(* Logix 5000 AddOnInstructionDefinition export Banner_Q4X_Param_v4; software revision 33.00; part 2 of 2 *)
(* tags used below, declared in another part *)
   Q4X : Banner_Q4X_v4;
   Port_Data : Banner_IOL_Port_v4;
   Port : INT;   // Enter the Port number that this AOI is to work with.
   Local_Control : DINT;
   Command_Being_Processed : BOOL;
   Update_Archive : BOOL;
   Index_Write_Inprocess : INT;
   Index_Write_Control : INT;
   Inprocess_Index : DINT;
(* Banner_Q4X_Param_v4, continued *)

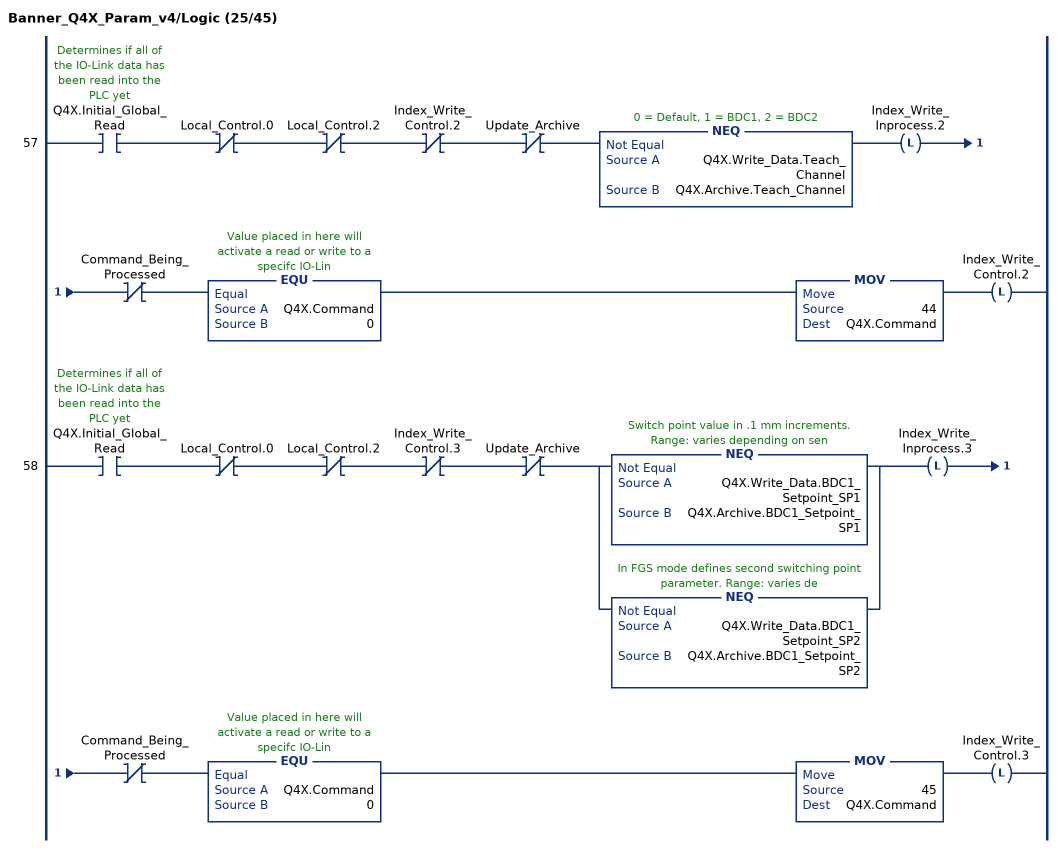
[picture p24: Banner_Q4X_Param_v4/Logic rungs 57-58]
   57: XIC(Q4X.Initial_Global_Read)XIO(Local_Control.0)XIO(Local_Control.2)XIO(Index_Write_Control.2)XIO(Update_Archive)NEQ(Q4X.Write_Data.Teach_Channel,Q4X.Archive.Teach_Channel)OTL(Index_Write_Inprocess.2)XIO(Command_Being_Processed)EQU(Q4X.Command,0)MOV(44,Q4X.Command)OTL(Index_Write_Control.2);
   58: XIC(Q4X.Initial_Global_Read)XIO(Local_Control.0)XIO(Local_Control.2)XIO(Index_Write_Control.3)XIO(Update_Archive)[NEQ(Q4X.Write_Data.BDC1_Setpoint_SP1,Q4X.Archive.BDC1_Setpoint_SP1) ,NEQ(Q4X.Write_Data.BDC1_Setpoint_SP2,Q4X.Archive.BDC1_Setpoint_SP2) ]OTL(Index_Write_Inprocess.3)XIO(Command_Being_Processed)EQU(Q4X.Command,0)MOV(45,Q4X.Command)OTL(Index_Write_Control.3);
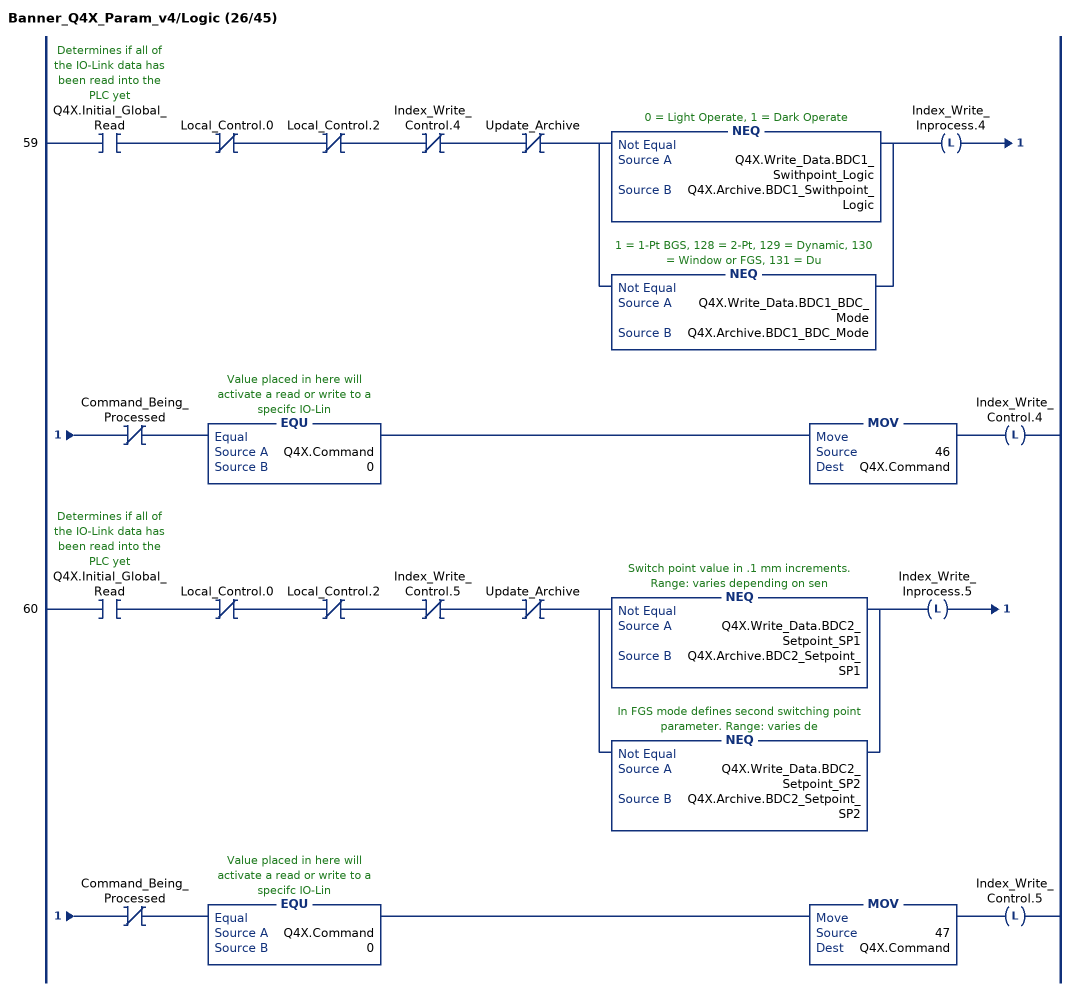
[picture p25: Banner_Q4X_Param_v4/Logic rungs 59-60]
   59: XIC(Q4X.Initial_Global_Read)XIO(Local_Control.0)XIO(Local_Control.2)XIO(Index_Write_Control.4)XIO(Update_Archive)[NEQ(Q4X.Write_Data.BDC1_Swithpoint_Logic,Q4X.Archive.BDC1_Swithpoint_Logic) ,NEQ(Q4X.Write_Data.BDC1_BDC_Mode,Q4X.Archive.BDC1_BDC_Mode) ]OTL(Index_Write_Inprocess.4)XIO(Command_Being_Processed)EQU(Q4X.Command,0)MOV(46,Q4X.Command)OTL(Index_Write_Control.4);
   60: XIC(Q4X.Initial_Global_Read)XIO(Local_Control.0)XIO(Local_Control.2)XIO(Index_Write_Control.5)XIO(Update_Archive)[NEQ(Q4X.Write_Data.BDC2_Setpoint_SP1,Q4X.Archive.BDC2_Setpoint_SP1) ,NEQ(Q4X.Write_Data.BDC2_Setpoint_SP2,Q4X.Archive.BDC2_Setpoint_SP2) ]OTL(Index_Write_Inprocess.5)XIO(Command_Being_Processed)EQU(Q4X.Command,0)MOV(47,Q4X.Command)OTL(Index_Write_Control.5);
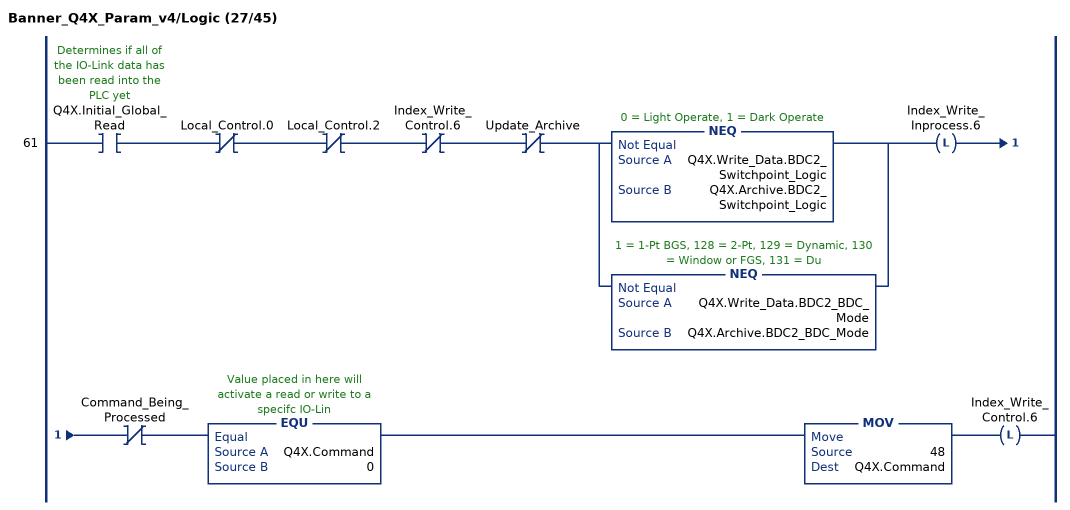
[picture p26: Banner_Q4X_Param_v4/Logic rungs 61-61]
   61: XIC(Q4X.Initial_Global_Read)XIO(Local_Control.0)XIO(Local_Control.2)XIO(Index_Write_Control.6)XIO(Update_Archive)[NEQ(Q4X.Write_Data.BDC2_Switchpoint_Logic,Q4X.Archive.BDC2_Switchpoint_Logic) ,NEQ(Q4X.Write_Data.BDC2_BDC_Mode,Q4X.Archive.BDC2_BDC_Mode) ]OTL(Index_Write_Inprocess.6)XIO(Command_Being_Processed)EQU(Q4X.Command,0)MOV(48,Q4X.Command)OTL(Index_Write_Control.6);
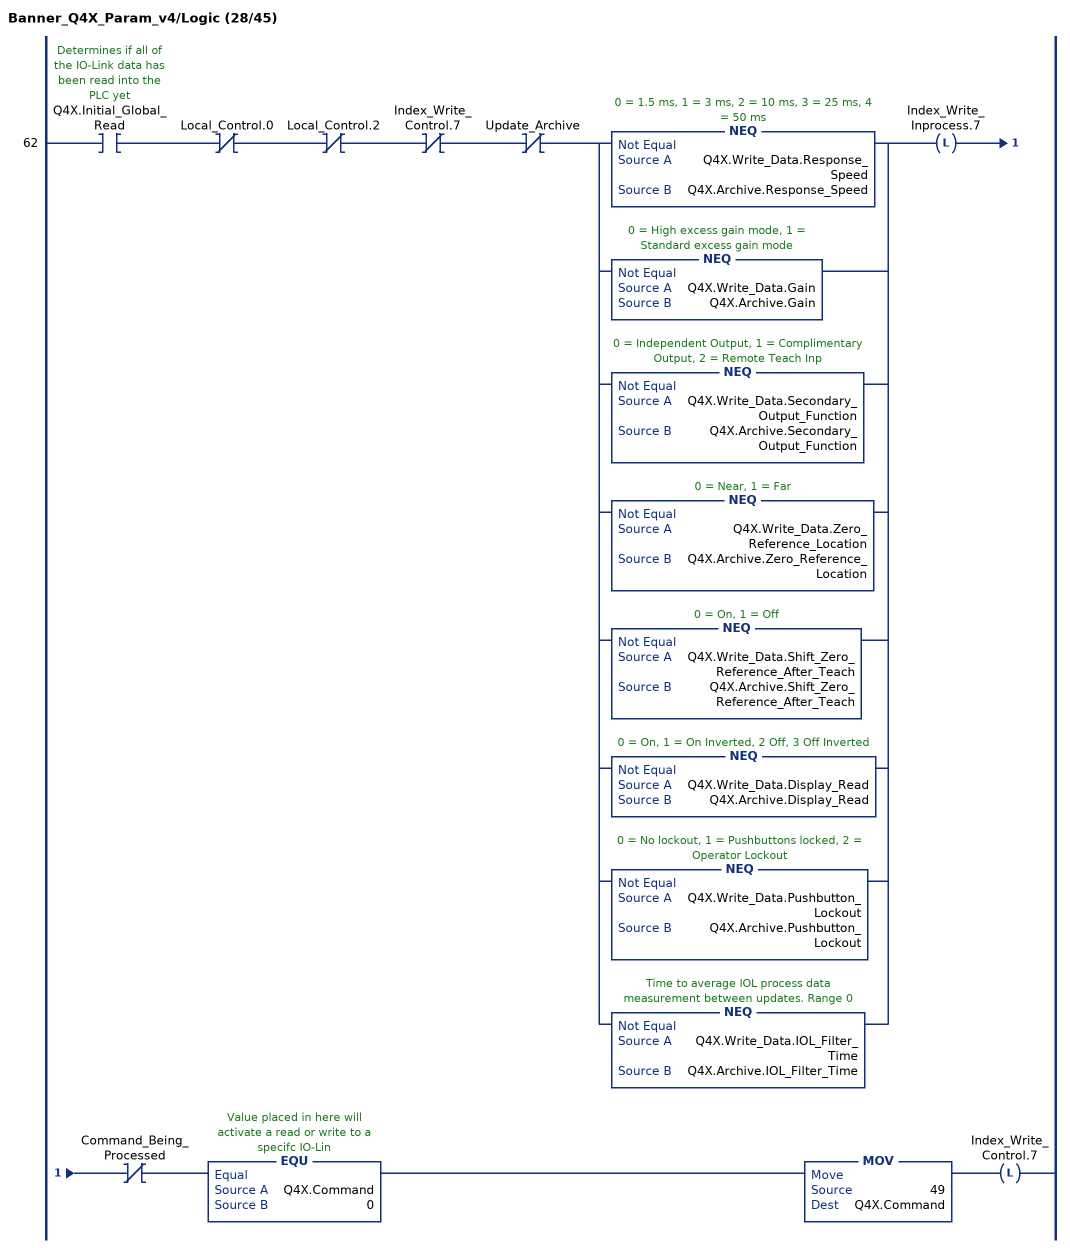
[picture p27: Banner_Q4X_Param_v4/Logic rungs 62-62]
   62: XIC(Q4X.Initial_Global_Read)XIO(Local_Control.0)XIO(Local_Control.2)XIO(Index_Write_Control.7)XIO(Update_Archive)[NEQ(Q4X.Write_Data.Response_Speed,Q4X.Archive.Response_Speed) ,NEQ(Q4X.Write_Data.Gain,Q4X.Archive.Gain) ,NEQ(Q4X.Write_Data.Secondary_Output_Function,Q4X.Archive.Secondary_Output_Function) ,NEQ(Q4X.Write_Data.Zero_Reference_Location,Q4X.Archive.Zero_Reference_Location) ,NEQ(Q4X.Write_Data.Shift_Zero_Reference_After_Teach,Q4X.Archive.Shift_Zero_Reference_After_Teach) ,NEQ(Q4X.Write_Data.Display_Read,Q4X.Archive.Display_Read) ,NEQ(Q4X.Write_Data.Pushbutton_Lockout,Q4X.Archive.Pushbutton_Lockout) ,NEQ(Q4X.Write_Data.IOL_Filter_Time,Q4X.Archive.IOL_Filter_Time) ]OTL(Index_Write_Inprocess.7)XIO(Command_Being_Processed)EQU(Q4X.Command,0)MOV(49,Q4X.Command)OTL(Index_Write_Control.7);
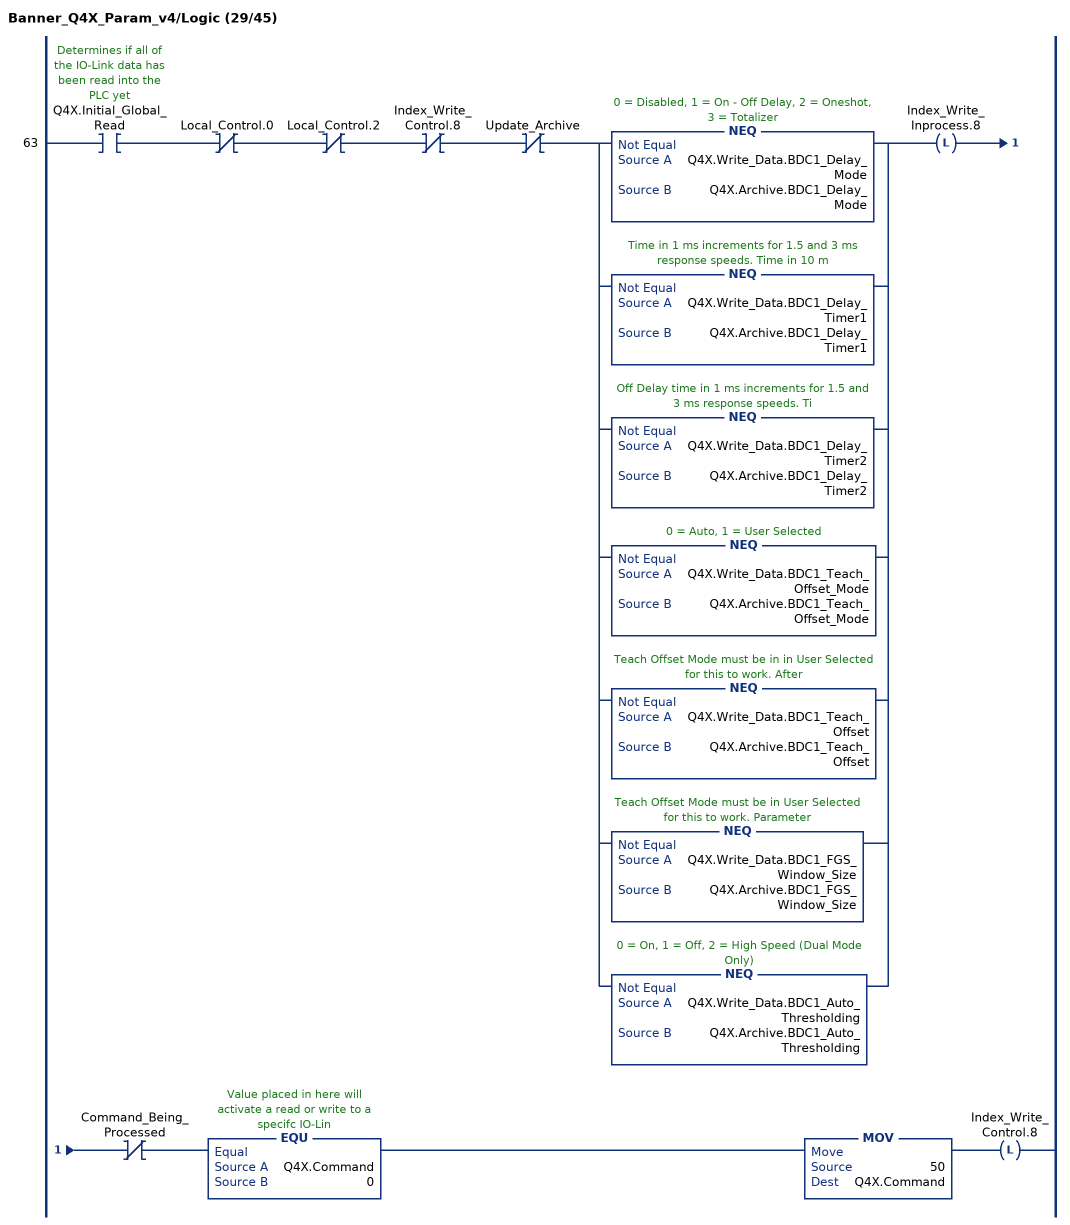
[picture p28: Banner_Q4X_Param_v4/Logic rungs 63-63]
   63: XIC(Q4X.Initial_Global_Read)XIO(Local_Control.0)XIO(Local_Control.2)XIO(Index_Write_Control.8)XIO(Update_Archive)[NEQ(Q4X.Write_Data.BDC1_Delay_Mode,Q4X.Archive.BDC1_Delay_Mode) ,NEQ(Q4X.Write_Data.BDC1_Delay_Timer1,Q4X.Archive.BDC1_Delay_Timer1) ,NEQ(Q4X.Write_Data.BDC1_Delay_Timer2,Q4X.Archive.BDC1_Delay_Timer2) ,NEQ(Q4X.Write_Data.BDC1_Teach_Offset_Mode,Q4X.Archive.BDC1_Teach_Offset_Mode) ,NEQ(Q4X.Write_Data.BDC1_Teach_Offset,Q4X.Archive.BDC1_Teach_Offset) ,NEQ(Q4X.Write_Data.BDC1_FGS_Window_Size,Q4X.Archive.BDC1_FGS_Window_Size) ,NEQ(Q4X.Write_Data.BDC1_Auto_Thresholding,Q4X.Archive.BDC1_Auto_Thresholding) ]OTL(Index_Write_Inprocess.8)XIO(Command_Being_Processed)EQU(Q4X.Command,0)MOV(50,Q4X.Command)OTL(Index_Write_Control.8);
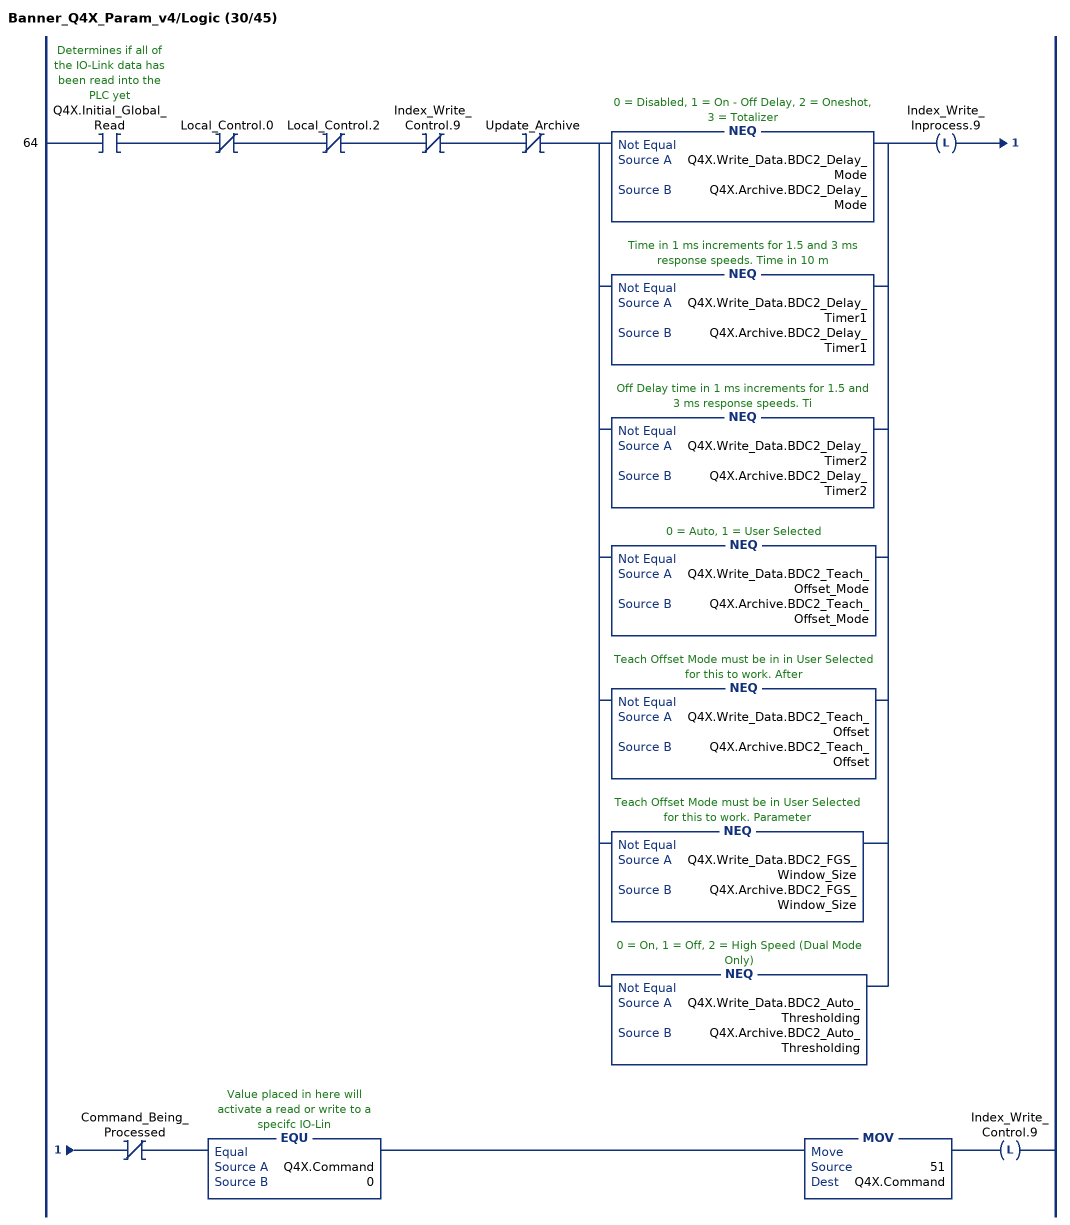
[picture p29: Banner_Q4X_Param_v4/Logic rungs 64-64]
   64: XIC(Q4X.Initial_Global_Read)XIO(Local_Control.0)XIO(Local_Control.2)XIO(Index_Write_Control.9)XIO(Update_Archive)[NEQ(Q4X.Write_Data.BDC2_Delay_Mode,Q4X.Archive.BDC2_Delay_Mode) ,NEQ(Q4X.Write_Data.BDC2_Delay_Timer1,Q4X.Archive.BDC2_Delay_Timer1) ,NEQ(Q4X.Write_Data.BDC2_Delay_Timer2,Q4X.Archive.BDC2_Delay_Timer2) ,NEQ(Q4X.Write_Data.BDC2_Teach_Offset_Mode,Q4X.Archive.BDC2_Teach_Offset_Mode) ,NEQ(Q4X.Write_Data.BDC2_Teach_Offset,Q4X.Archive.BDC2_Teach_Offset) ,NEQ(Q4X.Write_Data.BDC2_FGS_Window_Size,Q4X.Archive.BDC2_FGS_Window_Size) ,NEQ(Q4X.Write_Data.BDC2_Auto_Thresholding,Q4X.Archive.BDC2_Auto_Thresholding) ]OTL(Index_Write_Inprocess.9)XIO(Command_Being_Processed)EQU(Q4X.Command,0)MOV(51,Q4X.Command)OTL(Index_Write_Control.9);
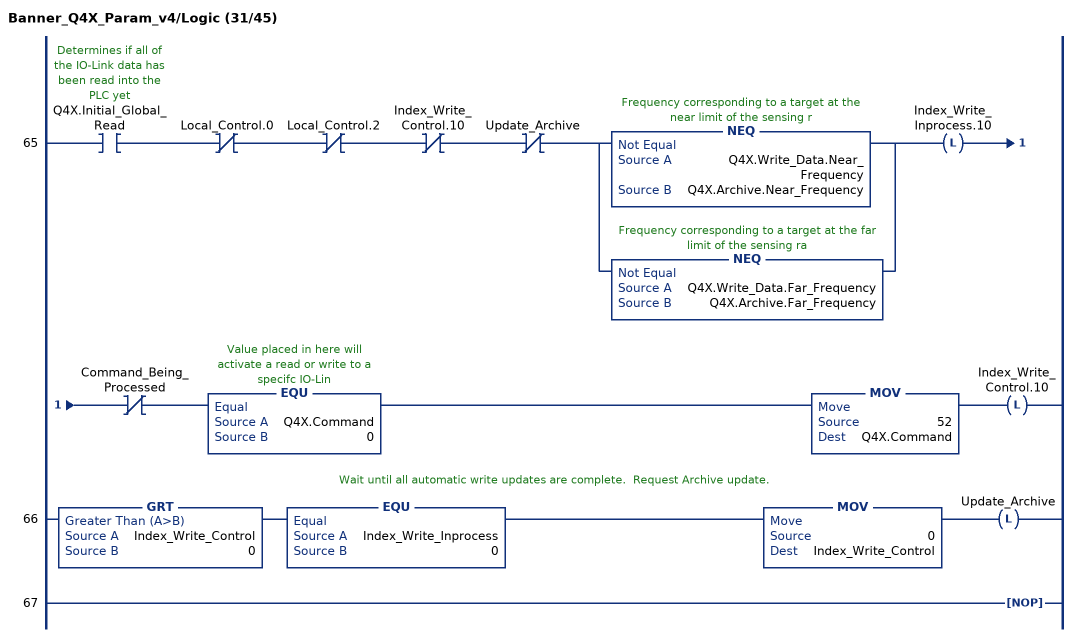
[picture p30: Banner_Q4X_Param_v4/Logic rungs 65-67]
   65: XIC(Q4X.Initial_Global_Read)XIO(Local_Control.0)XIO(Local_Control.2)XIO(Index_Write_Control.10)XIO(Update_Archive)[NEQ(Q4X.Write_Data.Near_Frequency,Q4X.Archive.Near_Frequency) ,NEQ(Q4X.Write_Data.Far_Frequency,Q4X.Archive.Far_Frequency) ]OTL(Index_Write_Inprocess.10)XIO(Command_Being_Processed)EQU(Q4X.Command,0)MOV(52,Q4X.Command)OTL(Index_Write_Control.10);
   // Wait until all automatic write updates are complete.  Request Archive update.
   66: GRT(Index_Write_Control,0)EQU(Index_Write_Inprocess,0)MOV(0,Index_Write_Control)OTL(Update_Archive);
   67: NOP();
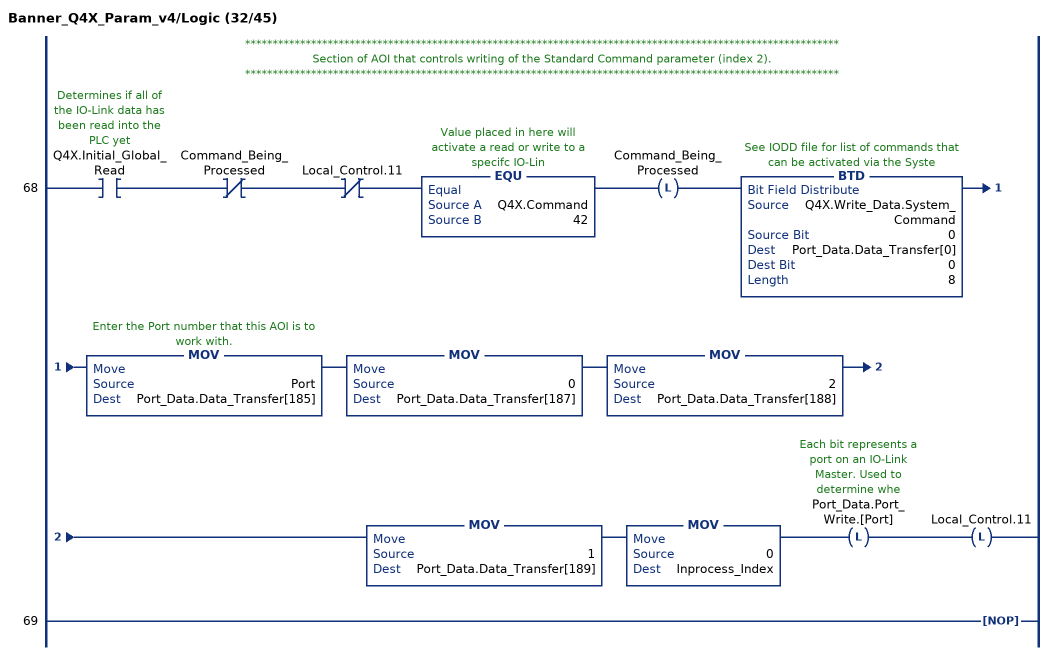
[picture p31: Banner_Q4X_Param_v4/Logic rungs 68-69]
   // ************************************************************************************************************
   // Section of AOI that controls writing of the Standard Command parameter (index 2).
   // ************************************************************************************************************
   68: XIC(Q4X.Initial_Global_Read)XIO(Command_Being_Processed)XIO(Local_Control.11)EQU(Q4X.Command,42)OTL(Command_Being_Processed)BTD(Q4X.Write_Data.System_Command,0,Port_Data.Data_Transfer[0],0,8)MOV(Port,Port_Data.Data_Transfer[185])MOV(0,Port_Data.Data_Transfer[187])MOV(2,Port_Data.Data_Transfer[188])MOV(1,Port_Data.Data_Transfer[189])MOV(0,Inprocess_Index)OTL(Port_Data.Port_Write.[Port])OTL(Local_Control.11);
   69: NOP();
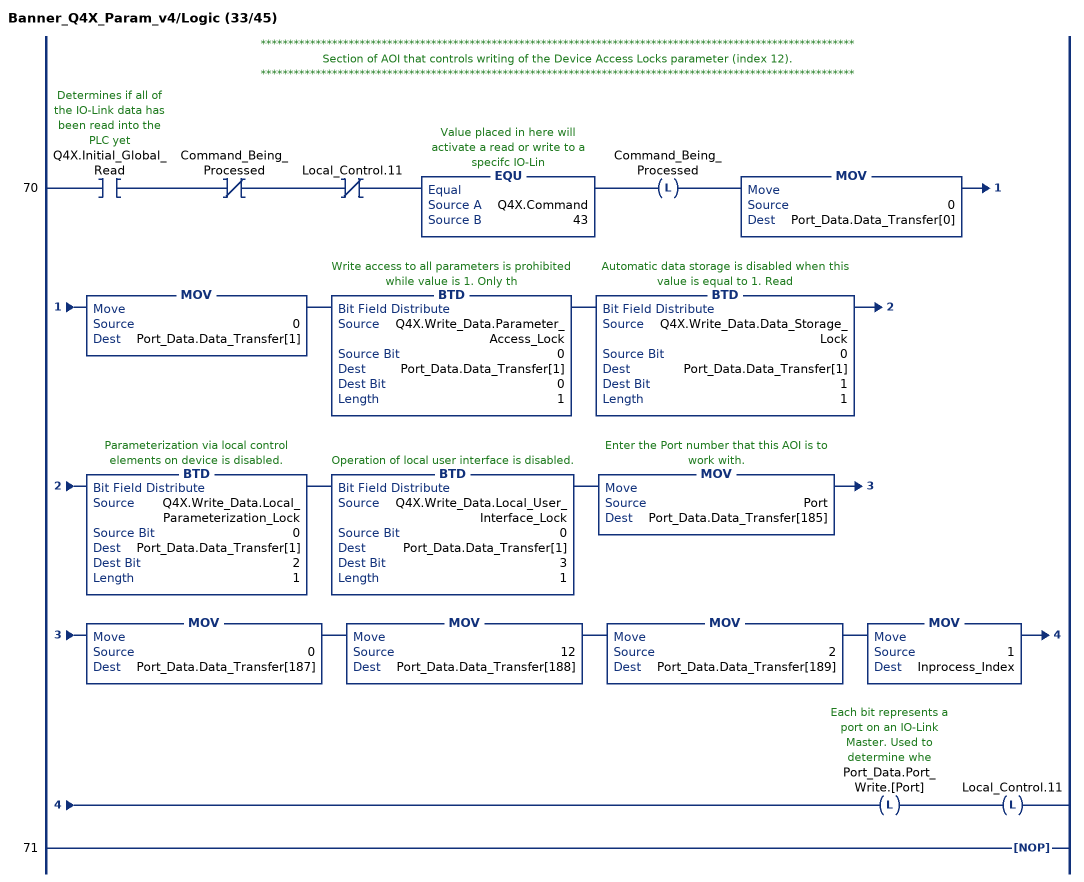
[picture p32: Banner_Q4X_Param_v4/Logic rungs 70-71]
   // ************************************************************************************************************
   // Section of AOI that controls writing of the Device Access Locks parameter (index 12).
   // ************************************************************************************************************
   70: XIC(Q4X.Initial_Global_Read)XIO(Command_Being_Processed)XIO(Local_Control.11)EQU(Q4X.Command,43)OTL(Command_Being_Processed)MOV(0,Port_Data.Data_Transfer[0])MOV(0,Port_Data.Data_Transfer[1])BTD(Q4X.Write_Data.Parameter_Access_Lock,0,Port_Data.Data_Transfer[1],0,1)BTD(Q4X.Write_Data.Data_Storage_Lock,0,Port_Data.Data_Transfer[1],1,1)BTD(Q4X.Write_Data.Local_Parameterization_Lock,0,Port_Data.Data_Transfer[1],2,1)BTD(Q4X.Write_Data.Local_User_Interface_Lock,0,Port_Data.Data_Transfer[1],3,1)MOV(Port,Port_Data.Data_Transfer[185])MOV(0,Port_Data.Data_Transfer[187])MOV(12,Port_Data.Data_Transfer[188])MOV(2,Port_Data.Data_Transfer[189])MOV(1,Inprocess_Index)OTL(Port_Data.Port_Write.[Port])OTL(Local_Control.11);
   71: NOP();
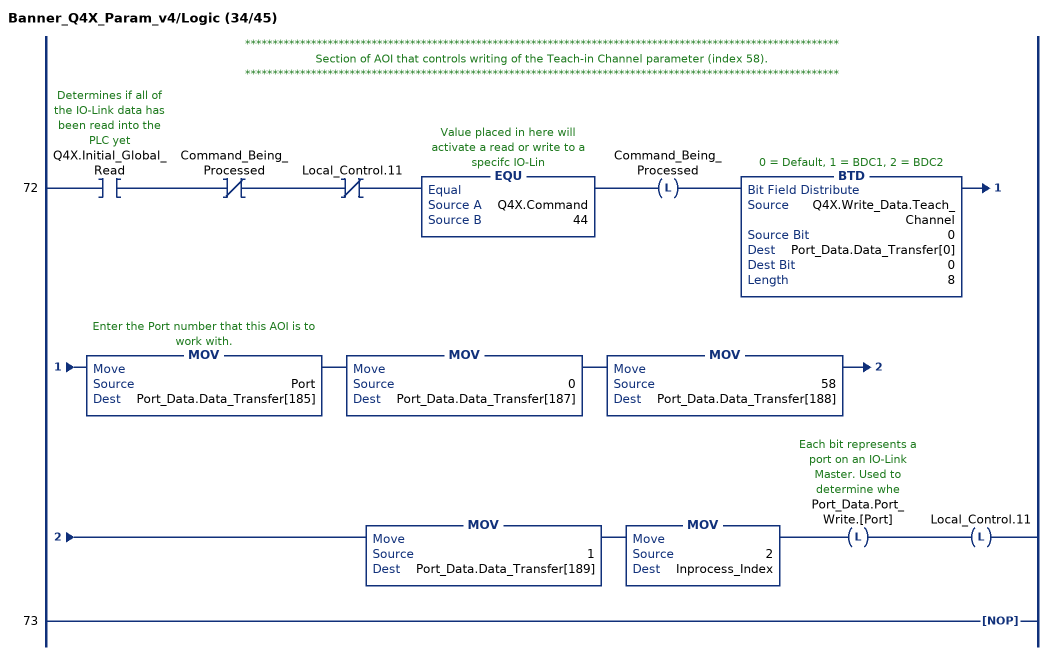
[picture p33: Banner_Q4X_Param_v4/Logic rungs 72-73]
   // ************************************************************************************************************
   // Section of AOI that controls writing of the Teach-in Channel parameter (index 58).
   // ************************************************************************************************************
   72: XIC(Q4X.Initial_Global_Read)XIO(Command_Being_Processed)XIO(Local_Control.11)EQU(Q4X.Command,44)OTL(Command_Being_Processed)BTD(Q4X.Write_Data.Teach_Channel,0,Port_Data.Data_Transfer[0],0,8)MOV(Port,Port_Data.Data_Transfer[185])MOV(0,Port_Data.Data_Transfer[187])MOV(58,Port_Data.Data_Transfer[188])MOV(1,Port_Data.Data_Transfer[189])MOV(2,Inprocess_Index)OTL(Port_Data.Port_Write.[Port])OTL(Local_Control.11);
   73: NOP();
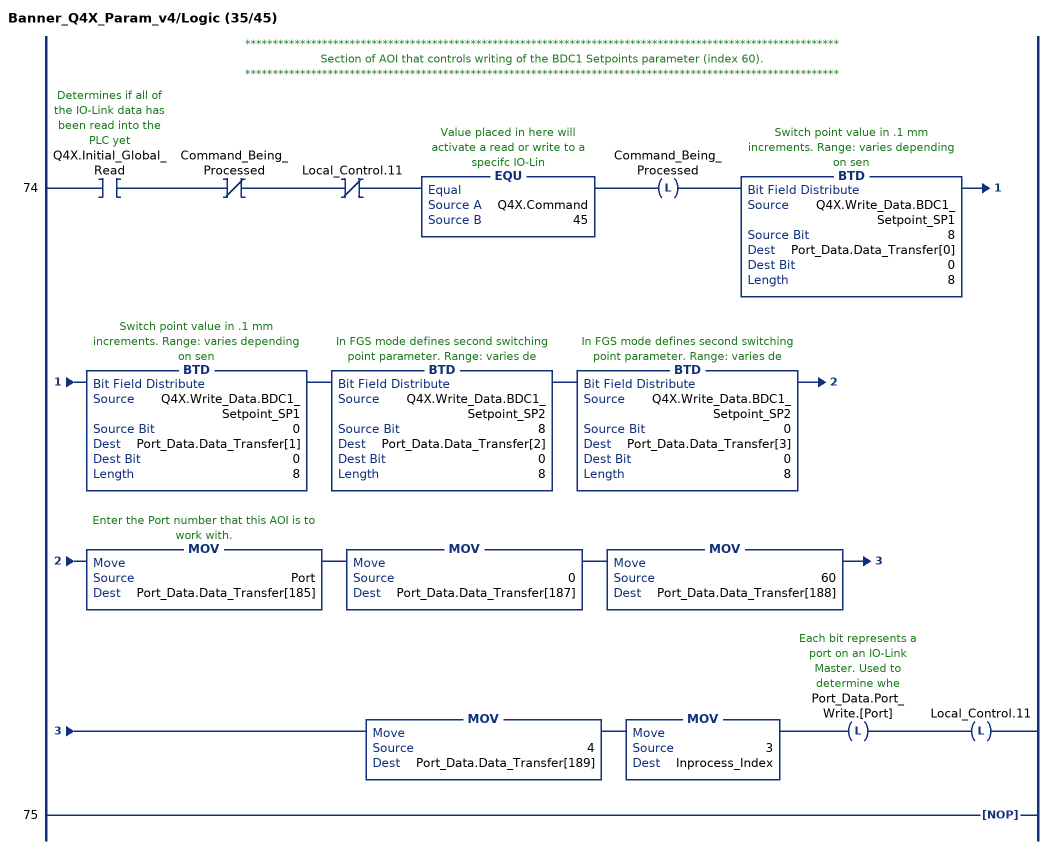
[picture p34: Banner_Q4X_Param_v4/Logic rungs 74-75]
   // ************************************************************************************************************
   // Section of AOI that controls writing of the BDC1 Setpoints parameter (index 60).
   // ************************************************************************************************************
   74: XIC(Q4X.Initial_Global_Read)XIO(Command_Being_Processed)XIO(Local_Control.11)EQU(Q4X.Command,45)OTL(Command_Being_Processed)BTD(Q4X.Write_Data.BDC1_Setpoint_SP1,8,Port_Data.Data_Transfer[0],0,8)BTD(Q4X.Write_Data.BDC1_Setpoint_SP1,0,Port_Data.Data_Transfer[1],0,8)BTD(Q4X.Write_Data.BDC1_Setpoint_SP2,8,Port_Data.Data_Transfer[2],0,8)BTD(Q4X.Write_Data.BDC1_Setpoint_SP2,0,Port_Data.Data_Transfer[3],0,8)MOV(Port,Port_Data.Data_Transfer[185])MOV(0,Port_Data.Data_Transfer[187])MOV(60,Port_Data.Data_Transfer[188])MOV(4,Port_Data.Data_Transfer[189])MOV(3,Inprocess_Index)OTL(Port_Data.Port_Write.[Port])OTL(Local_Control.11);
   75: NOP();
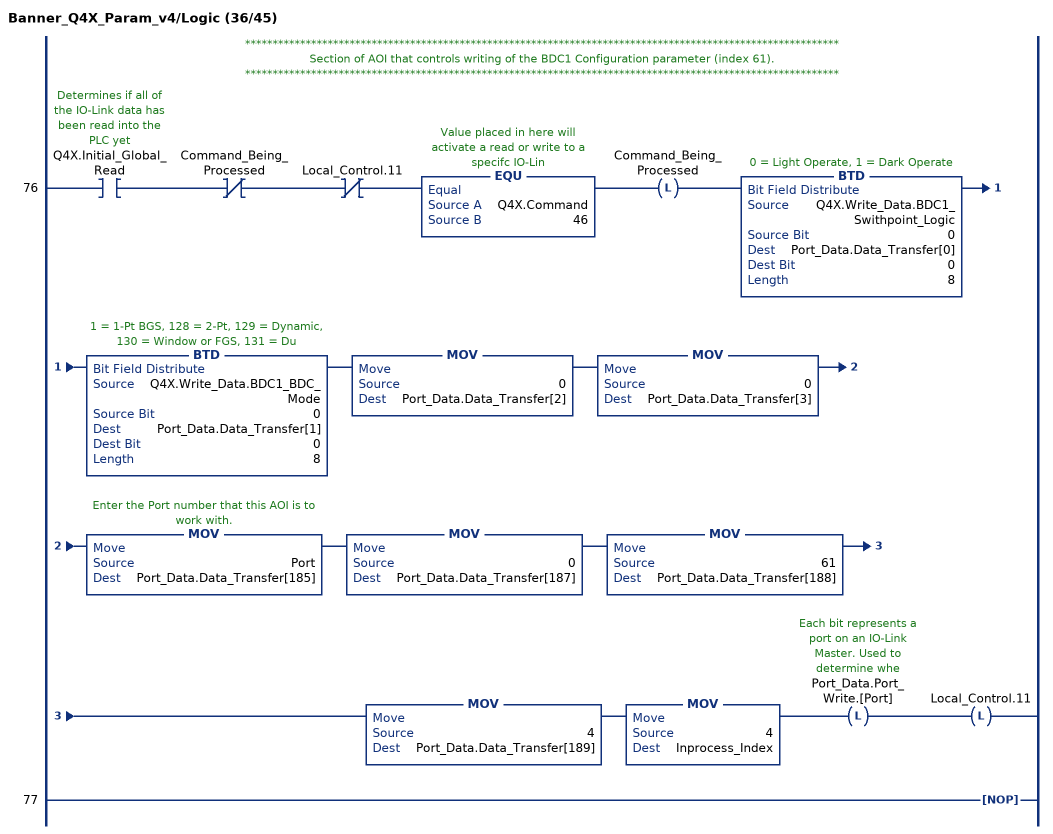
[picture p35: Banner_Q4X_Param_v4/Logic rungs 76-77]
   // ************************************************************************************************************
   // Section of AOI that controls writing of the BDC1 Configuration parameter (index 61).
   // ************************************************************************************************************
   76: XIC(Q4X.Initial_Global_Read)XIO(Command_Being_Processed)XIO(Local_Control.11)EQU(Q4X.Command,46)OTL(Command_Being_Processed)BTD(Q4X.Write_Data.BDC1_Swithpoint_Logic,0,Port_Data.Data_Transfer[0],0,8)BTD(Q4X.Write_Data.BDC1_BDC_Mode,0,Port_Data.Data_Transfer[1],0,8)MOV(0,Port_Data.Data_Transfer[2])MOV(0,Port_Data.Data_Transfer[3])MOV(Port,Port_Data.Data_Transfer[185])MOV(0,Port_Data.Data_Transfer[187])MOV(61,Port_Data.Data_Transfer[188])MOV(4,Port_Data.Data_Transfer[189])MOV(4,Inprocess_Index)OTL(Port_Data.Port_Write.[Port])OTL(Local_Control.11);
   77: NOP();
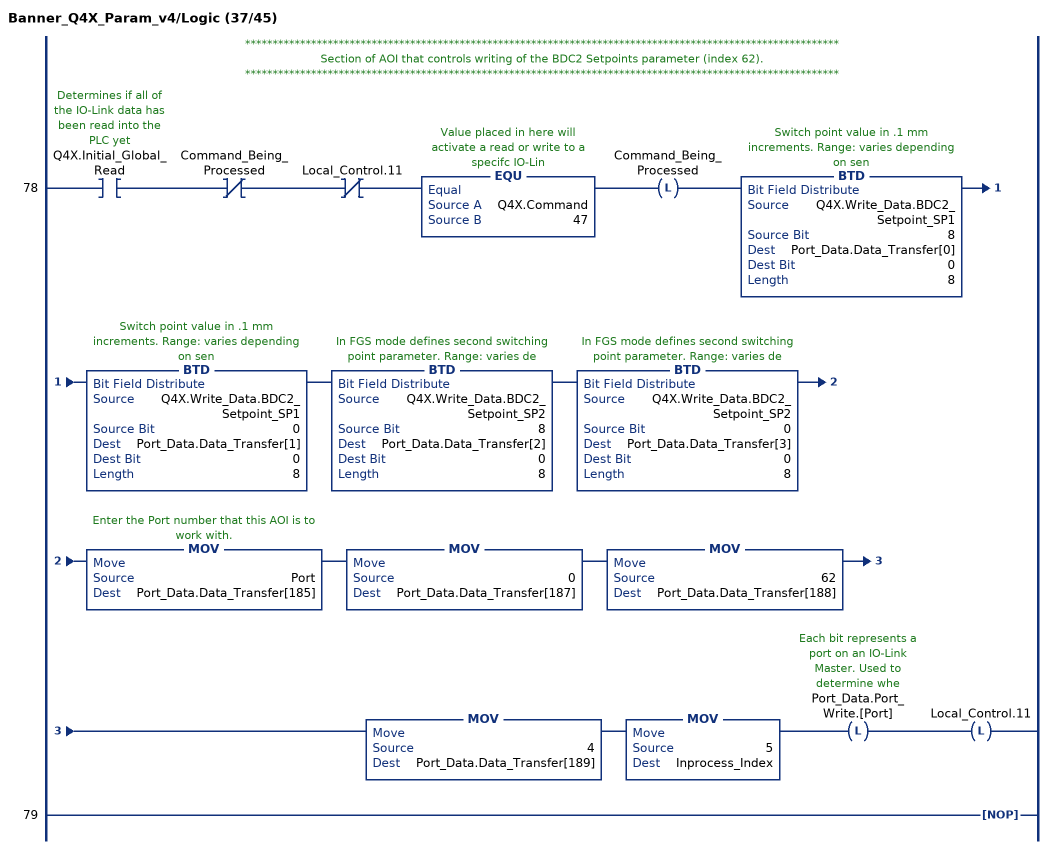
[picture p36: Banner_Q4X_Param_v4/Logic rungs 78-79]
   // ************************************************************************************************************
   // Section of AOI that controls writing of the BDC2 Setpoints parameter (index 62).
   // ************************************************************************************************************
   78: XIC(Q4X.Initial_Global_Read)XIO(Command_Being_Processed)XIO(Local_Control.11)EQU(Q4X.Command,47)OTL(Command_Being_Processed)BTD(Q4X.Write_Data.BDC2_Setpoint_SP1,8,Port_Data.Data_Transfer[0],0,8)BTD(Q4X.Write_Data.BDC2_Setpoint_SP1,0,Port_Data.Data_Transfer[1],0,8)BTD(Q4X.Write_Data.BDC2_Setpoint_SP2,8,Port_Data.Data_Transfer[2],0,8)BTD(Q4X.Write_Data.BDC2_Setpoint_SP2,0,Port_Data.Data_Transfer[3],0,8)MOV(Port,Port_Data.Data_Transfer[185])MOV(0,Port_Data.Data_Transfer[187])MOV(62,Port_Data.Data_Transfer[188])MOV(4,Port_Data.Data_Transfer[189])MOV(5,Inprocess_Index)OTL(Port_Data.Port_Write.[Port])OTL(Local_Control.11);
   79: NOP();
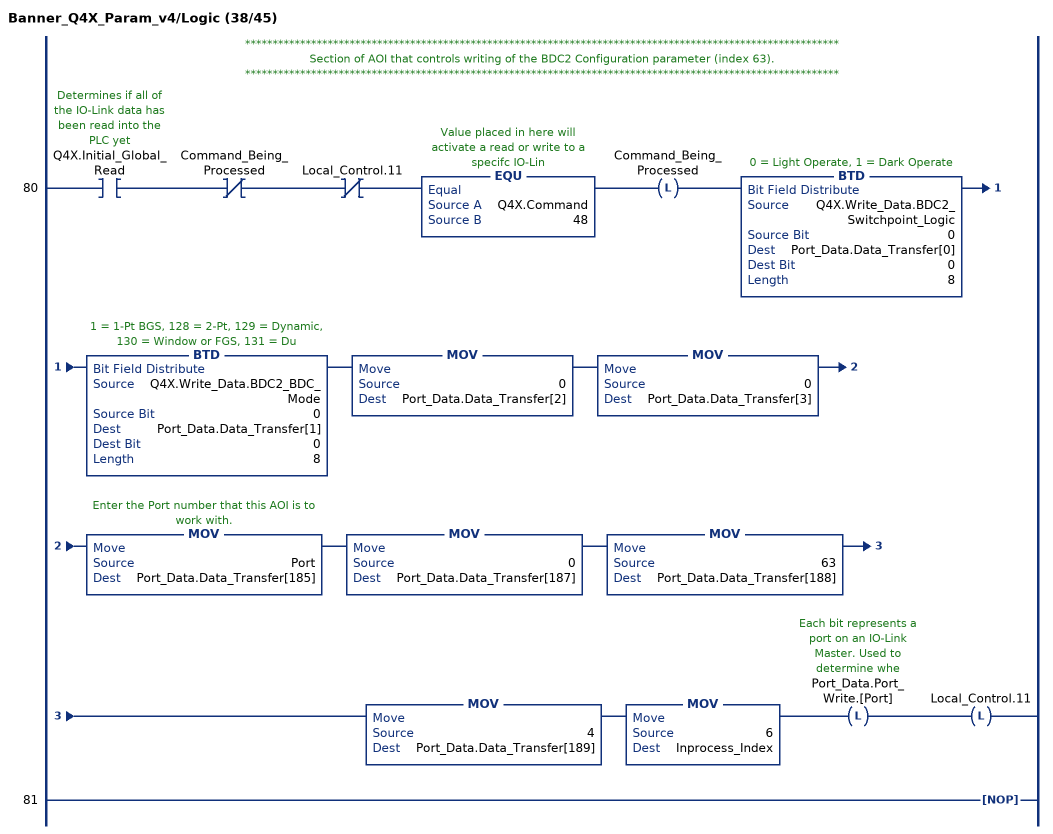
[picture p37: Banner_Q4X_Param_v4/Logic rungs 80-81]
   // ************************************************************************************************************
   // Section of AOI that controls writing of the BDC2 Configuration parameter (index 63).
   // ************************************************************************************************************
   80: XIC(Q4X.Initial_Global_Read)XIO(Command_Being_Processed)XIO(Local_Control.11)EQU(Q4X.Command,48)OTL(Command_Being_Processed)BTD(Q4X.Write_Data.BDC2_Switchpoint_Logic,0,Port_Data.Data_Transfer[0],0,8)BTD(Q4X.Write_Data.BDC2_BDC_Mode,0,Port_Data.Data_Transfer[1],0,8)MOV(0,Port_Data.Data_Transfer[2])MOV(0,Port_Data.Data_Transfer[3])MOV(Port,Port_Data.Data_Transfer[185])MOV(0,Port_Data.Data_Transfer[187])MOV(63,Port_Data.Data_Transfer[188])MOV(4,Port_Data.Data_Transfer[189])MOV(6,Inprocess_Index)OTL(Port_Data.Port_Write.[Port])OTL(Local_Control.11);
   81: NOP();
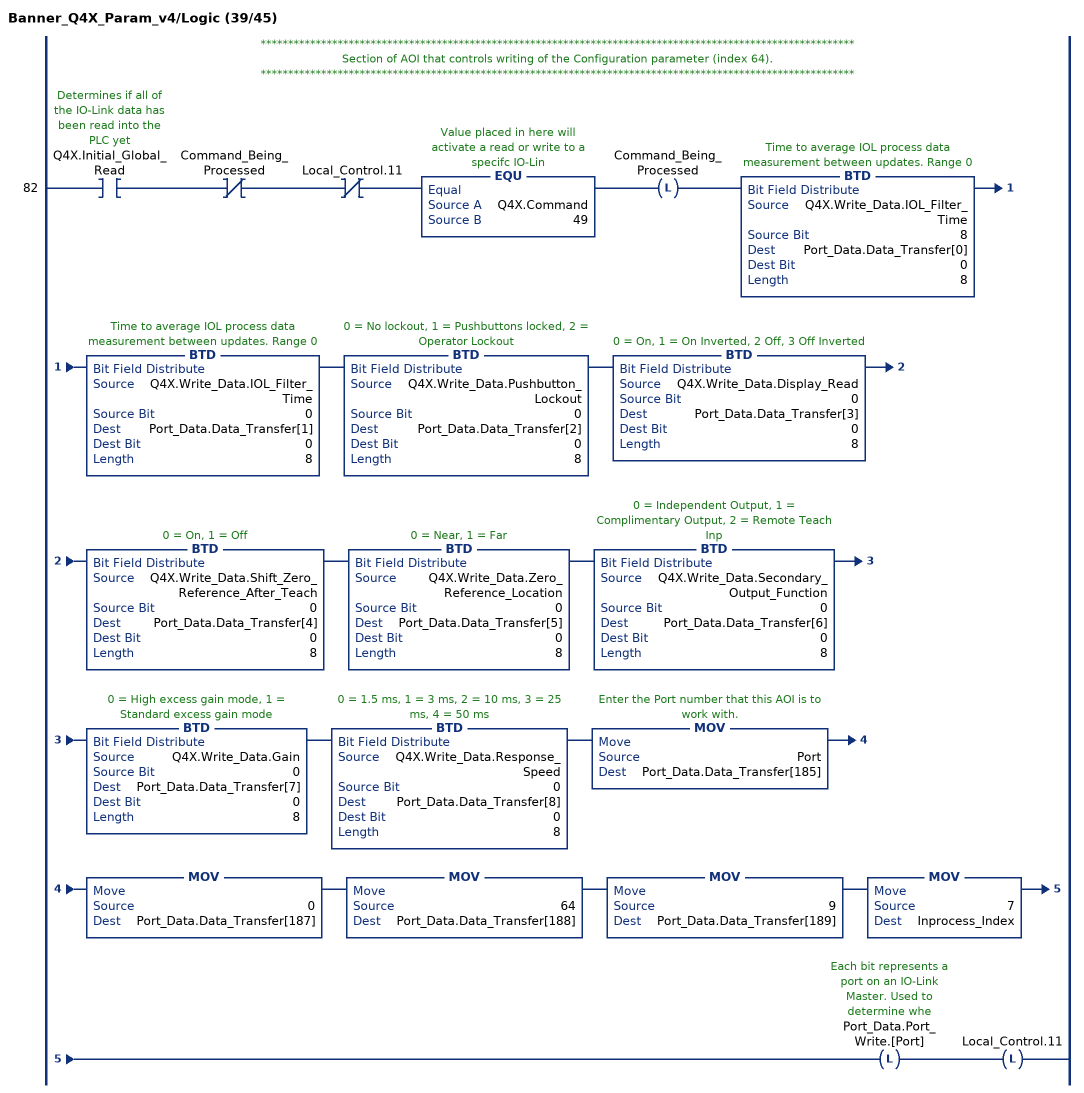
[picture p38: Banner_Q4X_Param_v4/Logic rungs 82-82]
   // ************************************************************************************************************
   // Section of AOI that controls writing of the Configuration parameter (index 64).
   // ************************************************************************************************************
   82: XIC(Q4X.Initial_Global_Read)XIO(Command_Being_Processed)XIO(Local_Control.11)EQU(Q4X.Command,49)OTL(Command_Being_Processed)BTD(Q4X.Write_Data.IOL_Filter_Time,8,Port_Data.Data_Transfer[0],0,8)BTD(Q4X.Write_Data.IOL_Filter_Time,0,Port_Data.Data_Transfer[1],0,8)BTD(Q4X.Write_Data.Pushbutton_Lockout,0,Port_Data.Data_Transfer[2],0,8)BTD(Q4X.Write_Data.Display_Read,0,Port_Data.Data_Transfer[3],0,8)BTD(Q4X.Write_Data.Shift_Zero_Reference_After_Teach,0,Port_Data.Data_Transfer[4],0,8)BTD(Q4X.Write_Data.Zero_Reference_Location,0,Port_Data.Data_Transfer[5],0,8)BTD(Q4X.Write_Data.Secondary_Output_Function,0,Port_Data.Data_Transfer[6],0,8)BTD(Q4X.Write_Data.Gain,0,Port_Data.Data_Transfer[7],0,8)BTD(Q4X.Write_Data.Response_Speed,0,Port_Data.Data_Transfer[8],0,8)MOV(Port,Port_Data.Data_Transfer[185])MOV(0,Port_Data.Data_Transfer[187])MOV(64,Port_Data.Data_Transfer[188])MOV(9,Port_Data.Data_Transfer[189])MOV(7,Inprocess_Index)OTL(Port_Data.Port_Write.[Port])OTL(Local_Control.11);
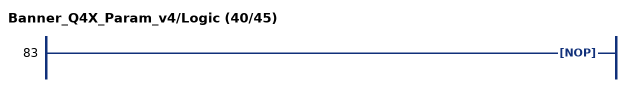
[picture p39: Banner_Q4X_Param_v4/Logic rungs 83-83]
   83: NOP();
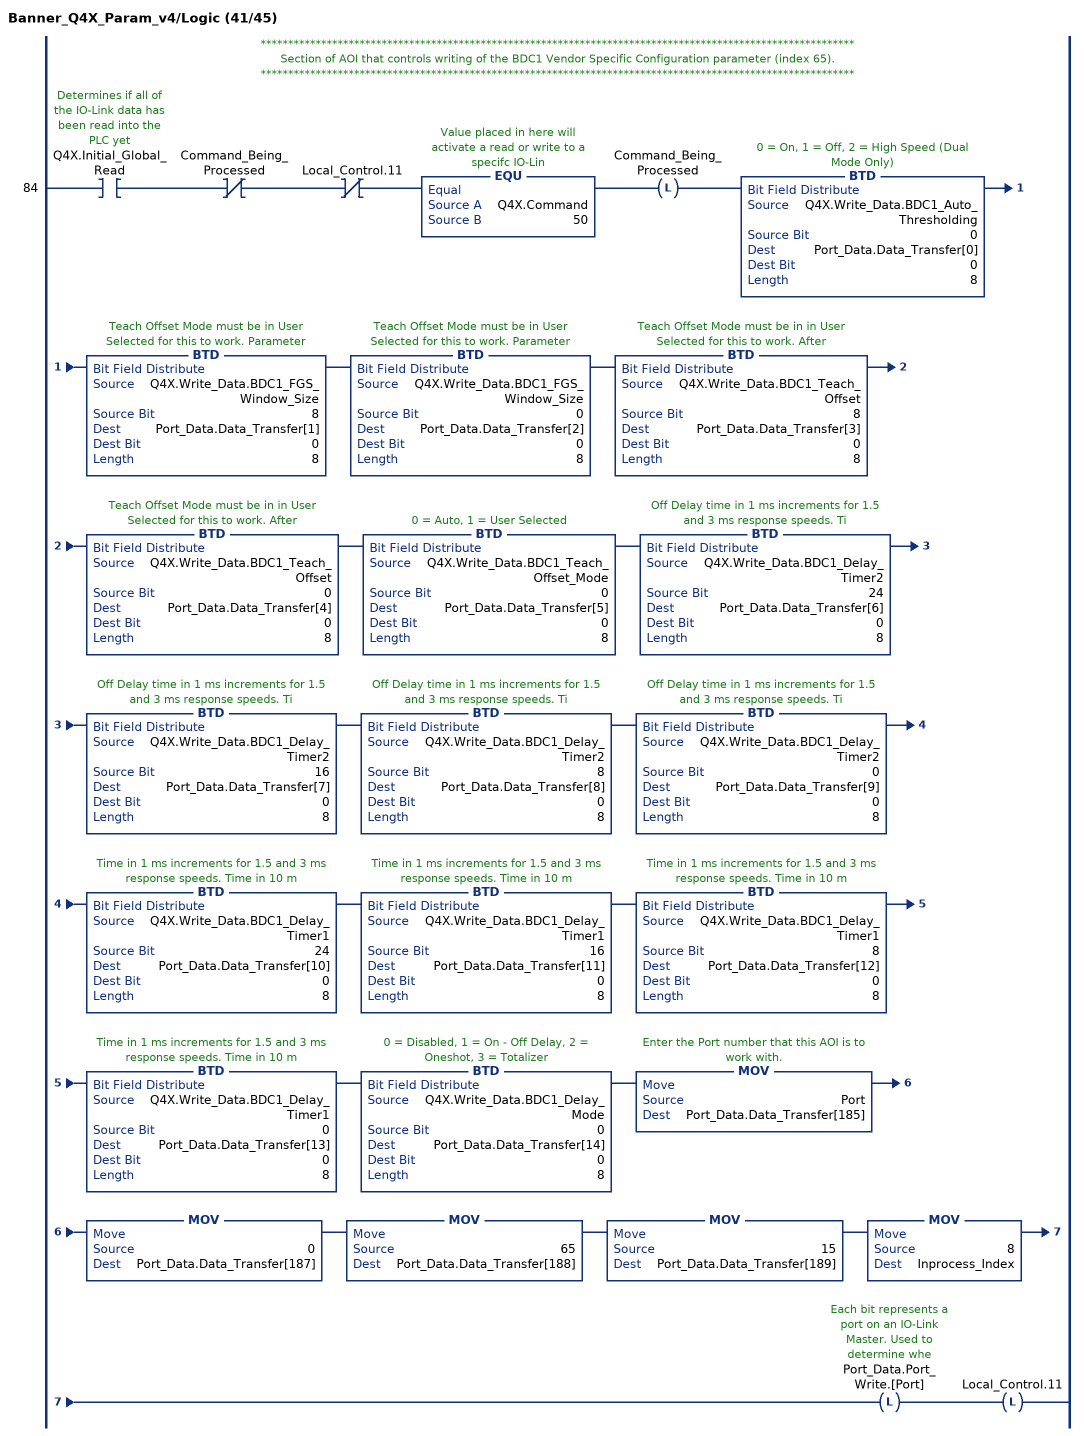
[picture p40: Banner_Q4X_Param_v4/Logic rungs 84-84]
   // ************************************************************************************************************
   // Section of AOI that controls writing of the BDC1 Vendor Specific Configuration parameter (index 65).
   // ************************************************************************************************************
   84: XIC(Q4X.Initial_Global_Read)XIO(Command_Being_Processed)XIO(Local_Control.11)EQU(Q4X.Command,50)OTL(Command_Being_Processed)BTD(Q4X.Write_Data.BDC1_Auto_Thresholding,0,Port_Data.Data_Transfer[0],0,8)BTD(Q4X.Write_Data.BDC1_FGS_Window_Size,8,Port_Data.Data_Transfer[1],0,8)BTD(Q4X.Write_Data.BDC1_FGS_Window_Size,0,Port_Data.Data_Transfer[2],0,8)BTD(Q4X.Write_Data.BDC1_Teach_Offset,8,Port_Data.Data_Transfer[3],0,8)BTD(Q4X.Write_Data.BDC1_Teach_Offset,0,Port_Data.Data_Transfer[4],0,8)BTD(Q4X.Write_Data.BDC1_Teach_Offset_Mode,0,Port_Data.Data_Transfer[5],0,8)BTD(Q4X.Write_Data.BDC1_Delay_Timer2,24,Port_Data.Data_Transfer[6],0,8)BTD(Q4X.Write_Data.BDC1_Delay_Timer2,16,Port_Data.Data_Transfer[7],0,8)BTD(Q4X.Write_Data.BDC1_Delay_Timer2,8,Port_Data.Data_Transfer[8],0,8)BTD(Q4X.Write_Data.BDC1_Delay_Timer2,0,Port_Data.Data_Transfer[9],0,8)BTD(Q4X.Write_Data.BDC1_Delay_Timer1,24,Port_Data.Data_Transfer[10],0,8)BTD(Q4X.Write_Data.BDC1_Delay_Timer1,16,Port_Data.Data_Transfer[11],0,8)BTD(Q4X.Write_Data.BDC1_Delay_Timer1,8,Port_Data.Data_Transfer[12],0,8)BTD(Q4X.Write_Data.BDC1_Delay_Timer1,0,Port_Data.Data_Transfer[13],0,8)BTD(Q4X.Write_Data.BDC1_Delay_Mode,0,Port_Data.Data_Transfer[14],0,8)MOV(Port,Port_Data.Data_Transfer[185])MOV(0,Port_Data.Data_Transfer[187])MOV(65,Port_Data.Data_Transfer[188])MOV(15,Port_Data.Data_Transfer[189])MOV(8,Inprocess_Index)OTL(Port_Data.Port_Write.[Port])OTL(Local_Control.11);
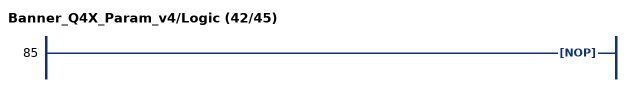
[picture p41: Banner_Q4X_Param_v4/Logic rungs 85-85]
   85: NOP();
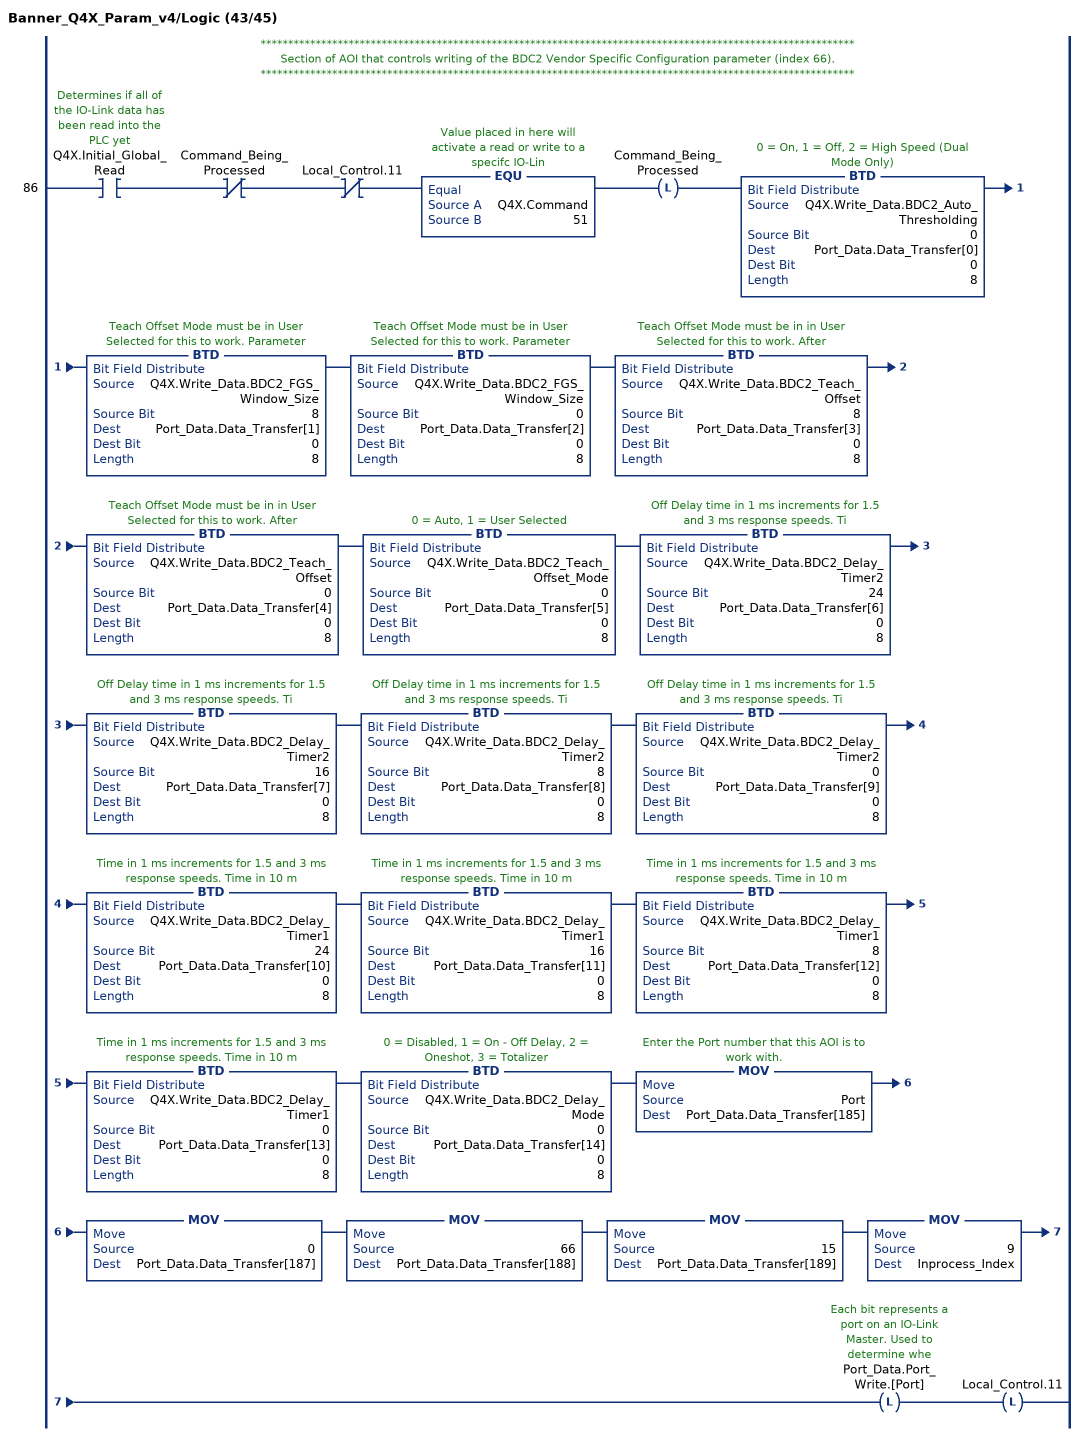
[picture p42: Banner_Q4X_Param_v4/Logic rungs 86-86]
   // ************************************************************************************************************
   // Section of AOI that controls writing of the BDC2 Vendor Specific Configuration parameter (index 66).
   // ************************************************************************************************************
   86: XIC(Q4X.Initial_Global_Read)XIO(Command_Being_Processed)XIO(Local_Control.11)EQU(Q4X.Command,51)OTL(Command_Being_Processed)BTD(Q4X.Write_Data.BDC2_Auto_Thresholding,0,Port_Data.Data_Transfer[0],0,8)BTD(Q4X.Write_Data.BDC2_FGS_Window_Size,8,Port_Data.Data_Transfer[1],0,8)BTD(Q4X.Write_Data.BDC2_FGS_Window_Size,0,Port_Data.Data_Transfer[2],0,8)BTD(Q4X.Write_Data.BDC2_Teach_Offset,8,Port_Data.Data_Transfer[3],0,8)BTD(Q4X.Write_Data.BDC2_Teach_Offset,0,Port_Data.Data_Transfer[4],0,8)BTD(Q4X.Write_Data.BDC2_Teach_Offset_Mode,0,Port_Data.Data_Transfer[5],0,8)BTD(Q4X.Write_Data.BDC2_Delay_Timer2,24,Port_Data.Data_Transfer[6],0,8)BTD(Q4X.Write_Data.BDC2_Delay_Timer2,16,Port_Data.Data_Transfer[7],0,8)BTD(Q4X.Write_Data.BDC2_Delay_Timer2,8,Port_Data.Data_Transfer[8],0,8)BTD(Q4X.Write_Data.BDC2_Delay_Timer2,0,Port_Data.Data_Transfer[9],0,8)BTD(Q4X.Write_Data.BDC2_Delay_Timer1,24,Port_Data.Data_Transfer[10],0,8)BTD(Q4X.Write_Data.BDC2_Delay_Timer1,16,Port_Data.Data_Transfer[11],0,8)BTD(Q4X.Write_Data.BDC2_Delay_Timer1,8,Port_Data.Data_Transfer[12],0,8)BTD(Q4X.Write_Data.BDC2_Delay_Timer1,0,Port_Data.Data_Transfer[13],0,8)BTD(Q4X.Write_Data.BDC2_Delay_Mode,0,Port_Data.Data_Transfer[14],0,8)MOV(Port,Port_Data.Data_Transfer[185])MOV(0,Port_Data.Data_Transfer[187])MOV(66,Port_Data.Data_Transfer[188])MOV(15,Port_Data.Data_Transfer[189])MOV(9,Inprocess_Index)OTL(Port_Data.Port_Write.[Port])OTL(Local_Control.11);
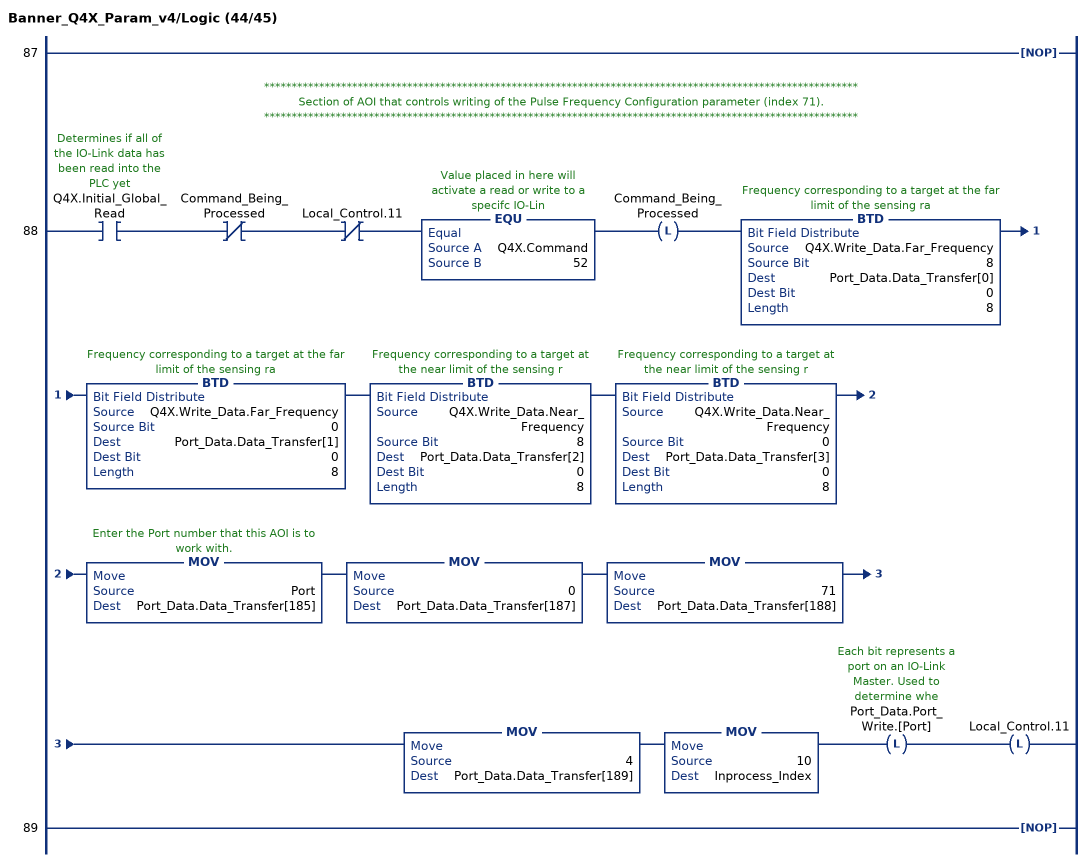
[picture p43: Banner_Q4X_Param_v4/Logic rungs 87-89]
   87: NOP();
   // ************************************************************************************************************
   // Section of AOI that controls writing of the Pulse Frequency Configuration parameter (index 71).
   // ************************************************************************************************************
   88: XIC(Q4X.Initial_Global_Read)XIO(Command_Being_Processed)XIO(Local_Control.11)EQU(Q4X.Command,52)OTL(Command_Being_Processed)BTD(Q4X.Write_Data.Far_Frequency,8,Port_Data.Data_Transfer[0],0,8)BTD(Q4X.Write_Data.Far_Frequency,0,Port_Data.Data_Transfer[1],0,8)BTD(Q4X.Write_Data.Near_Frequency,8,Port_Data.Data_Transfer[2],0,8)BTD(Q4X.Write_Data.Near_Frequency,0,Port_Data.Data_Transfer[3],0,8)MOV(Port,Port_Data.Data_Transfer[185])MOV(0,Port_Data.Data_Transfer[187])MOV(71,Port_Data.Data_Transfer[188])MOV(4,Port_Data.Data_Transfer[189])MOV(10,Inprocess_Index)OTL(Port_Data.Port_Write.[Port])OTL(Local_Control.11);
   89: NOP();
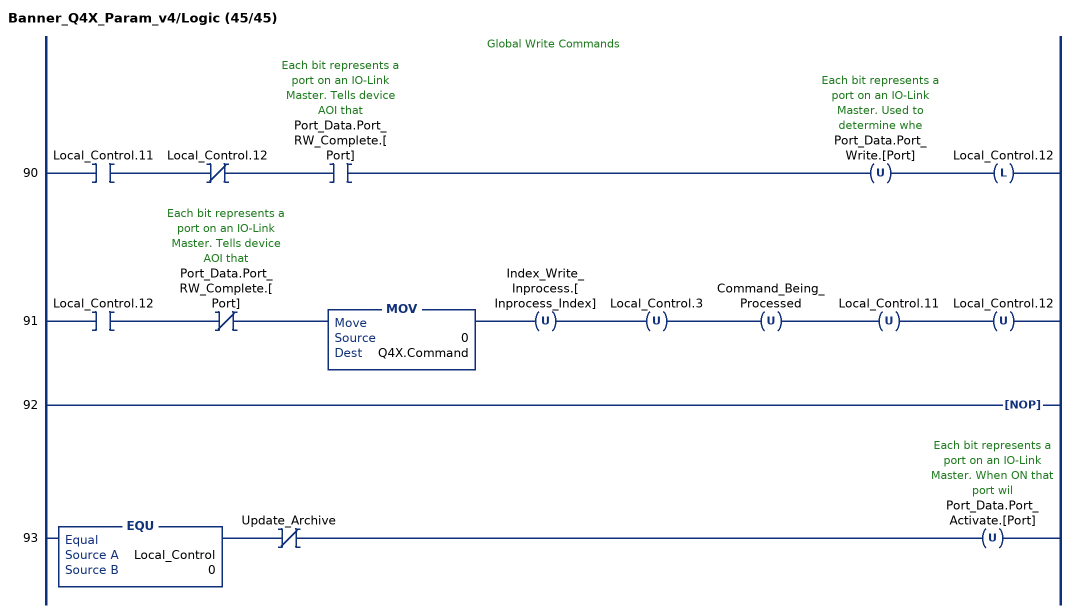
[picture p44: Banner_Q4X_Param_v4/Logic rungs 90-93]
   // Global Write Commands
   90: XIC(Local_Control.11)XIO(Local_Control.12)XIC(Port_Data.Port_RW_Complete.[Port])OTU(Port_Data.Port_Write.[Port])OTL(Local_Control.12);
   91: XIC(Local_Control.12)XIO(Port_Data.Port_RW_Complete.[Port])MOV(0,Q4X.Command)OTU(Index_Write_Inprocess.[Inprocess_Index])OTU(Local_Control.3)OTU(Command_Being_Processed)OTU(Local_Control.11)OTU(Local_Control.12);
   92: NOP();
   93: EQU(Local_Control,0)XIO(Update_Archive)OTU(Port_Data.Port_Activate.[Port]);
END_ROUTINE
END_ADD_ON_INSTRUCTION
